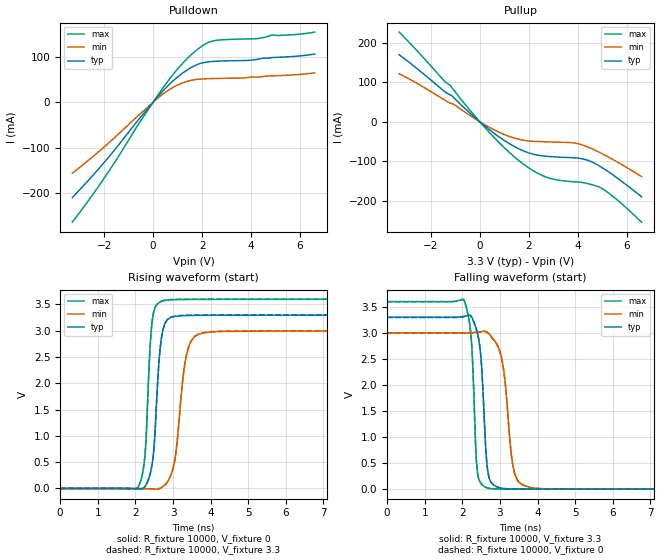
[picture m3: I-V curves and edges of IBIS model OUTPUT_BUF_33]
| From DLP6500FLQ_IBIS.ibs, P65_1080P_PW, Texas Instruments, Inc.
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[Model]   OUTPUT_BUF_33
Model_type  Output
Vref =   0
Rref =   10000
Cref =   0p
Vmeas =   1.5
| variable   typ   min   max
C_comp   2.74pF   0.97pF   4.36pF
| C_pullup   3.23pF   1.86pF   4.36pF
| C_pulldown   2.25pF   0.97pF   3.53pF
[Temperature Range]   40   140   -40
| Ambient temperature   25   125   -40
[Voltage range]   3.3   3   3.6
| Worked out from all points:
|   slope of the pulldown table from 0 to 0.495 V, typ, clamps not added: 16.4 ohm
|   slope of the pullup table from 0 to 0.495 V, typ, clamps not added: 19.8 ohm
|   rising waveform, R_fixture 10000, V_fixture 0: 20-80 % time 175ps typ, 261ps min, 144ps max; typ from 0 V to 3.29 V
|   falling waveform, R_fixture 10000, V_fixture 3.3: 20-80 % time 154ps typ, 240ps min, 124ps max; typ from 3.3 V to 0 V
|   rising waveform, R_fixture 10000, V_fixture 3.3: 20-80 % time 175ps typ, 260ps min, 144ps max; typ from 0 V to 3.3 V
|   falling waveform, R_fixture 10000, V_fixture 0: 20-80 % time 154ps typ, 240ps min, 124ps max; typ from 3.29 V to 0 V
[Pulldown]
| OUTPUT_BUF_33
|   Voltage   I(typ)   I(min)   I(max)
-3.3V     -210.2mA   -156.5mA   -264.6mA
-1.935V   -128.7mA   -95.54mA   -162.5mA
-575mV    -37mA      -28.06mA   -46.34mA
400mV     24.83mA    18.02mA    31.6mA
1.115V    60.74mA    40.78mA    80.43mA
1.815V    83.36mA    50.51mA    116.7mA
2.215V    88.88mA    51.89mA    130.9mA
2.56V     90.43mA    52.46mA    136.3mA
4.205V    94.18mA    55.66mA    140.3mA
4.885V    98.64mA    58.28mA    148.4mA
5.705V    100.9mA    60.31mA    148.9mA
6.6V      106.4mA    64.82mA    154.8mA
[Pullup]
| OUTPUT_BUF_33
|   Voltage   I(typ)   I(min)   I(max)
-3.3V     170.4mA    121.8mA    227.6mA
-1.455V   77.36mA    55.91mA    103.6mA
-1.215V   68.42mA    47.69mA    92.44mA
390mV     -19.96mA   -14.03mA   -27.09mA
1.65V     -69.98mA   -45.01mA   -101.1mA
2.24V     -82.76mA   -49.4mA    -126.2mA
2.78V     -87.35mA   -50.72mA   -141.5mA
3.835V    -90.93mA   -53.29mA   -151.8mA
4.45V     -98.3mA    -64.83mA   -157.3mA
4.87V     -111.6mA   -76.89mA   -165.1mA
5.195V    -124.4mA   -87.38mA   -177.6mA
6.6V      -189.7mA   -138.6mA   -254.2mA
[Ramp]
| OUTPUT_BUF_33
| variable   typ   min   max
dV/dt_r   1.98/1.78E-10   1.80/2.66E-10   2.16/1.48E-10
dV/dt_f   2.00/1.61E-10   1.82/2.49E-10   2.19/1.28E-10
R_load = 10000
[Rising Waveform]
| OUTPUT_BUF_33
R_fixture =   10000
C_fixture =   0
L_fixture =   0
V_fixture =   0
V_fixture_min = 0
V_fixture_max = 0
|   Time   V(typ)   V(min)   V(max)
0s        1.24nV     2.096nV    979.1pV
2.08ns    -9.32mV    -91.77uV   35.94mV
2.255ns   40.58mV    -3.024mV   632.2mV
2.45ns    484.2mV    -9.562mV   3.197V
2.64ns    2.518V     -1.534mV   3.536V
2.765ns   3.091V     56mV       3.57V
3.05ns    3.27V      543.8mV    3.589V
3.38ns    3.287V     2.597V     3.592V
3.82ns    3.291V     2.957V     3.594V
23ns      3.294V     2.993V     3.595V
[Falling Waveform]
| OUTPUT_BUF_33
R_fixture =   10000
C_fixture =   0
L_fixture =   0
V_fixture =   3.3
V_fixture_min = 3
V_fixture_max = 3.6
|   Time   V(typ)   V(min)   V(max)
0s        3.3V       3V         3.6V
2.05ns    3.318V     3V         3.624V
2.235ns   3.321V     3.004V     2.916V
2.37ns    3.083V     3.014V     625.4mV
2.445ns   2.848V     3.019V     184.9mV
2.705ns   246mV      2.987V     17.08mV
3.07ns    16.08mV    2.428V     2.205mV
3.39ns    4.343mV    310.7mV    345.1uV
3.825ns   492.4uV    29.57mV    111.1uV
23ns      1.414uV    1.998uV    415.8nV
[Rising Waveform]
| OUTPUT_BUF_33
R_fixture =   10000
C_fixture =   0
L_fixture =   0
V_fixture =   3.3
V_fixture_min = 3
V_fixture_max = 3.6
|   Time   V(typ)   V(min)   V(max)
0s        1.242nV    2.1nV      980.3pV
2.08ns    -9.333mV   -91.86uV   35.98mV
2.255ns   40.63mV    -3.029mV   633.3mV
2.45ns    485.2mV    -9.579mV   3.203V
2.64ns    2.525V     -1.547mV   3.542V
2.765ns   3.098V     56.1mV     3.575V
3.05ns    3.277V     545.6mV    3.594V
3.375ns   3.293V     2.593V     3.598V
3.775ns   3.297V     2.958V     3.599V
23ns      3.3V       3V         3.6V
[Falling Waveform]
| OUTPUT_BUF_33
R_fixture =   10000
C_fixture =   0
L_fixture =   0
V_fixture =   0
V_fixture_min = 0
V_fixture_max = 0
|   Time   V(typ)   V(min)   V(max)
0s        3.294V     2.993V     3.595V
2.05ns    3.312V     2.992V     3.618V
2.235ns   3.314V     2.996V     2.908V
2.37ns    3.074V     3.006V     619.8mV
2.445ns   2.838V     3.011V     183.9mV
2.705ns   243.6mV    2.979V     16.99mV
3.07ns    15.94mV    2.413V     2.192mV
3.39ns    4.31mV     302.8mV    342.4uV
3.81ns    519.3uV    31.49mV    111.9uV
23ns      1.41uV     1.99uV     415.2nV
